(* Logix 5000 Routine export PassthroughMsg; software revision 24.00 *)

TYPE DNetPassThroughRequest :
STRUCT
   Node : SINT;   // Target DeviceNet Node
   Service : INT;   // CIP Service
   Class : INT;   // CIP Class Id
   Instance : INT;   // CIP Instance Id
   Attribute : INT;   // CIP Attribute Id
   DataSize : INT;   // Request Data Size (bytes)
   Data : SINT[256];   // Request Data
END_STRUCT
END_TYPE

TYPE DNetPassThroughResponse :
STRUCT
   Status : INT;   // Status
   ServiceResponse : SINT;   // CIP Service Response
   DNetStatus : SINT;   // Target DeviceNet Status
   DataSize : INT;   // Response Data Size (bytes)
   Data : SINT[256];   // Response Data
END_STRUCT
END_TYPE

VAR_GLOBAL   (* controller tags *)
   PassThroughMessage : MESSAGE;
        MessageParameters(MessageType := CIP Generic, RequestedLength := 270, ConnectedFlag := 2, ConnectionPath := Eth, 2, 192.168.1.147, ServiceCode := 16#006b, ObjectType := 16#0436, TargetObject := 1, LocalElement := PassThroughRequest, DestinationTag := PassThroughResponse)
   PassThroughResponse : DNetPassThroughResponse;
   PassThroughTrigger : BOOL;
   PassThroughRequest : DNetPassThroughRequest := (Node := 16#04, Service := 16#000e, Class := 16#0001, Instance := 1, Attribute := 3);
END_VAR

PROGRAM MainProgram

ROUTINE PassthroughMsg   (* ladder *)
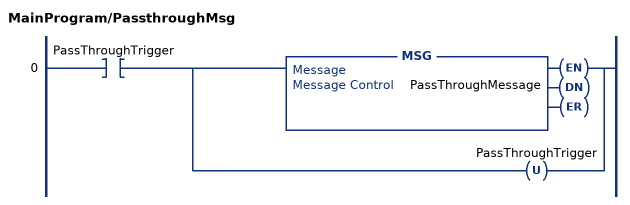
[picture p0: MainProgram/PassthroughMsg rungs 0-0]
   0: XIC(PassThroughTrigger)[MSG(PassThroughMessage) ,OTU(PassThroughTrigger) ];
END_ROUTINE
END_PROGRAM
